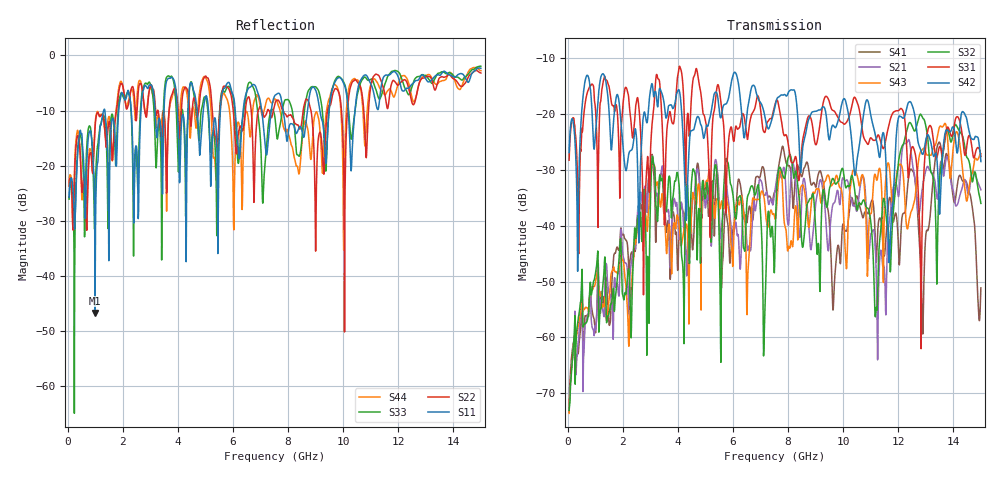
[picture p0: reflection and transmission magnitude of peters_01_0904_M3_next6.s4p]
# MHZ S RI R 50.00
! FREQ  S11  S12  S13  S14
!  S21  S22  S23  S24
!  S31  S32  S33  S34
!  S41  S42  S43  S44
!  REAL  IMAG  REAL  IMAG  REAL  IMAG  REAL  IMAG
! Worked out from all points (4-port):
!   1496 points, 50 MHz to 15 GHz, reference 50 ohm
!   strongest paths, dB at 50 MHz, 3.79 GHz, 7.53 GHz, 11.27 GHz, 15 GHz:
!     S42: -26.9, -18.9, -18.6, -26.4, -28.6
!     S31: -28.3, -21.6, -18.3, -23.8, -27.6
!     S32: -73.0, -36.5, -42.5, -48.6, -36.0
!     S43: -73.6, -45.8, -38.9, -30.7, -27.1
!     S21: -73.3, -38.6, -33.5, -55.7, -33.6
!     S41: -72.8, -39.1, -33.8, -39.9, -51.1
!   lowest |S11| = -46.7 dB at 990 MHz (marker M1), VSWR 1.01, Z = 49.8 + j0.424 ohm
!   |S11| at or under -10 dB: start of sweep to 1.304 GHz; 1.346 GHz to 1.851 GHz (504.8 MHz wide, 31.6 % of centre); 7.821 GHz to 8.704 GHz (882.5 MHz wide, 10.7 % of centre)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
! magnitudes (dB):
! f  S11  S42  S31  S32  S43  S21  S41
! 50 MHz  -25.8  -26.9  -28.3  -73.0  -73.6  -73.3  -72.8
! 990 MHz  -46.7  -24.6  -18.3  -49.0  -50.6  -57.9  -58.1
! 7.8 GHz  -9.4  -16.7  -22.7  -30.9  -33.4  -30.5  -25.8
! 11.19 GHz  -8.8  -24.4  -24.6  -55.0  -31.4  -46.9  -46.0
! 12.88 GHz  -3.5  -27.3  -37.3  -20.7  -26.4  -33.2  -58.3
! 13.49 GHz  -3.6  -37.5  -26.0  -32.7  -22.5  -31.1  -25.1
! 15 GHz  -2.3  -28.6  -27.6  -36.0  -27.1  -33.6  -51.1
